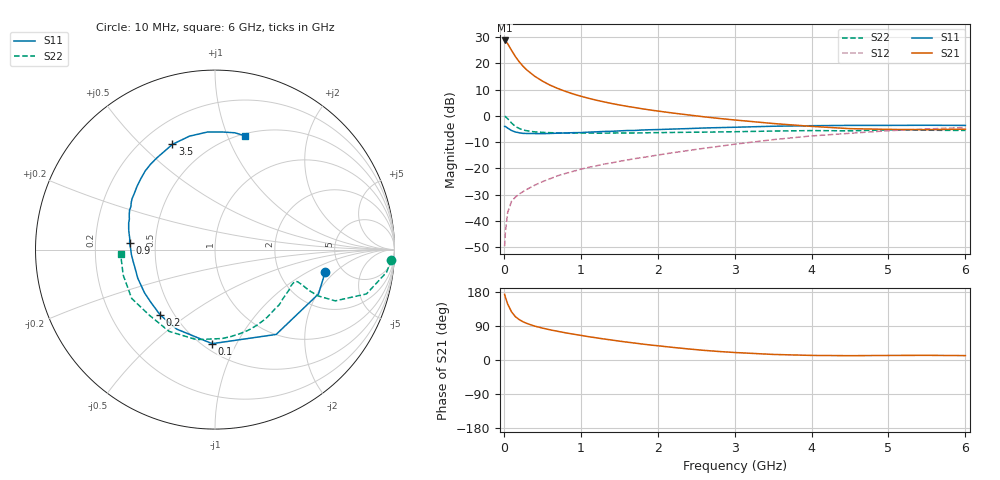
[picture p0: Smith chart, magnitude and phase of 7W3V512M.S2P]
! Infineon Technologies  Discrete & RF Semiconductors
! BFS17W
! Si NPN RF Bipolar Junction Transistor in SOT323
! VCE = 3.5 V  IC = 12 mA
! Common Emitter S-Parameters:  August  1999
# GHz  S  MA  R  50
!  f  S11  S21  S12  S22
! GHz  MAG  ANG  MAG  ANG  MAG  ANG  MAG  ANG
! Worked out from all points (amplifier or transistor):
!   36 points, 10 MHz to 6 GHz, reference 50 ohm
!   highest |S21| = 28.7 dB at 10 MHz (marker M1)
!   |S21| within 3 dB of that: start of sweep to 84.89 MHz
!   unconditionally stable (mu >= 1): 364.8 MHz to 2.419 GHz; 4.686 GHz to end of sweep
!   at 250 MHz: K = 0.85, MSG = 23.9 dB, |S12| = -28.9 dB
!   at 1.4 GHz: K = 1.20, MAG = 8.6 dB, |S12| = -17.9 dB
!   at 6 GHz: K = 1.06, MAG = -1.9 dB, |S12| = -4.5 dB
!   S11 on the Smith chart (normalised r, x): 10 MHz: 3.68, -1.53; 100 MHz: 0.56, -0.80; 200 MHz: 0.42, -0.39; 900 MHz: 0.35, +0.03; 3.5 GHz: 0.32, +0.63; 6 GHz: 0.52, +1.16
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0.01  0.6266 -11.6  27.15 173.2  0.0033 79.7  0.9841 -3.3
0.02  0.6273 -23.2  26.61 165.9  0.0061 81.7  0.9644 -7.5
0.05  0.5827 -54.2  23.53 147.5  0.0145 70.1  0.8795 -16.3
0.1  0.5243 -91.7  17.61 127.0  0.0236 58.7  0.7281 -23.1
0.15  0.4917 -115.7  13.4 114.4  0.0283 53.9  0.6279 -24.2
0.2  0.4749 -130.2  10.66 106.6  0.0325 55.9  0.5733 -23.5
0.25  0.4625 -140.8  8.763 100.8  0.036 56.1  0.5382 -22.5
0.3  0.4607 -148.5  7.426 96.4  0.0398 57.5  0.5187 -21.9
0.4  0.4589 -159.6  5.678 89.5  0.0476 60.7  0.4941 -21.3
0.5  0.4571 -166.6  4.585 84.3  0.0556 62.2  0.4839 -21.5
0.6  0.4611 -172.1  3.836 79.7  0.0633 64.2  0.4772 -22.3
0.7  0.4665 -176.6  3.317 75.7  0.0722 65.7  0.473 -23.6
0.9  0.4769 175.7  2.605 68.4  0.0874 66.8  0.4678 -27.0
1.1  0.4885 168.9  2.155 61.6  0.1042 67.2  0.4677 -31.3
1.3  0.5034 162.8  1.841 55.5  0.1203 67.8  0.4669 -36.2
1.6  0.5241 155.3  1.514 47.2  0.1436 68.5  0.4696 -43.8
2.2  0.5592 141.0  1.127 33.2  0.1984 69.1  0.4818 -61.1
2.8  0.5956 127.2  0.89 22.4  0.2628 66.9  0.4923 -79.5
3.5  0.6326 112.0  0.713 14.7  0.3515 61.5  0.5121 -101.7
4.5  0.6566 93.6  0.569 11.4  0.4645 48.9  0.5173 -135.2
5.5  0.6603 80.3  0.544 12.3  0.5612 36.3  0.5309 -164.5
6  0.6552 75.3  0.556 11.6  0.5988 30.1  0.5264 -177.3
